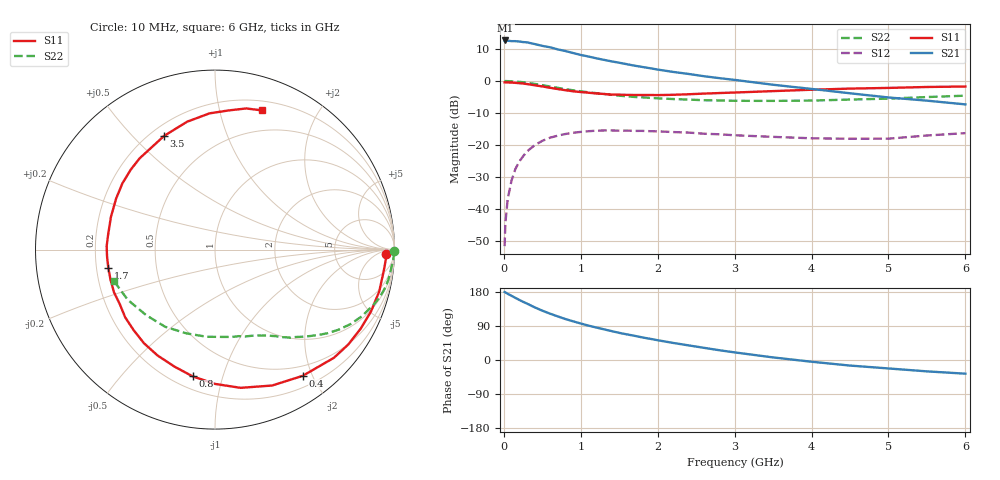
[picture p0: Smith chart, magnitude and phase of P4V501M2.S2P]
! SIEMENS Small Signal Semiconductors
! BFP182
! Si NPN RF Bipolar Junction Transistor in SOT143
! VCE = 0.5 V  IC = 1.2 mA
! Common Emitter S-Parameters:  March  1996
# GHz  S  MA  R  50
!  f  S11  S21  S12  S22
! GHz  MAG  ANG  MAG  ANG  MAG  ANG  MAG  ANG
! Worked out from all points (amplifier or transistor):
!   36 points, 10 MHz to 6 GHz, reference 50 ohm
!   highest |S21| = 12.7 dB at 20 MHz (marker M1)
!   |S21| within 3 dB of that: start of sweep to 740.6 MHz
!   unconditionally stable (mu >= 1): 2.31 GHz to end of sweep
!   at 250 MHz: K = 0.11, MSG = 17.9 dB, |S12| = -23.6 dB
!   at 1.4 GHz: K = 0.62, MSG = 10.8 dB, |S12| = -15.5 dB
!   at 6 GHz: K = 1.39, MAG = 0.8 dB, |S12| = -16.3 dB
!   S11 on the Smith chart (normalised r, x): 10 MHz: 33, -16; 400 MHz: 0.35, -1.86; 800 MHz: 0.28, -0.80; 1.7 GHz: 0.25, -0.08; 3.5 GHz: 0.25, +0.62; 6 GHz: 0.29, +1.36
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0.01  0.9518 -1.4  4.228 179.3  0.0026 87.4  0.995 -0.6
0.02  0.954 -3.0  4.306 178.5  0.0059 88.5  0.9977 -1.4
0.05  0.9476 -7.2  4.265 174.7  0.0142 87.6  0.9942 -3.3
0.1  0.9444 -14.3  4.198 169.4  0.0277 81.6  0.9863 -6.5
0.15  0.9349 -21.6  4.198 164.0  0.0419 76.3  0.9806 -9.9
0.25  0.9115 -35.5  4.065 153.6  0.0663 68.1  0.9557 -16.1
0.3  0.8958 -42.3  4.022 149.0  0.0788 64.1  0.9373 -18.9
0.4  0.8564 -55.2  3.784 139.0  0.0988 56.0  0.8997 -24.3
0.5  0.8215 -67.2  3.542 130.2  0.1157 49.0  0.8607 -28.9
0.6  0.7833 -79.5  3.368 122.3  0.1294 43.1  0.82 -33.0
0.8  0.7171 -100.0  2.944 108.1  0.148 32.3  0.7456 -39.7
0.9  0.6899 -109.1  2.739 102.1  0.1548 27.8  0.7145 -42.4
1.1  0.6548 -127.2  2.414 90.7  0.1636 20.2  0.6646 -47.1
1.4  0.6115 -150.0  2.027 76.3  0.1684 10.6  0.6089 -53.3
1.7  0.6032 -170.2  1.735 63.8  0.1655 4.1  0.5618 -58.4
1.9  0.6039 178.1  1.584 56.0  0.1638 0.4  0.544 -61.8
2.2  0.6076 162.7  1.386 45.1  0.1587 -3.8  0.5215 -67.1
2.8  0.6473 136.4  1.108 25.8  0.1465 -9.5  0.4959 -78.9
3.5  0.6941 114.1  0.873 6.8  0.1335 -10.9  0.4879 -95.5
4.5  0.7597 92.3  0.642 -14.7  0.1247 -7.0  0.512 -122.9
5.5  0.8055 77.5  0.492 -30.0  0.1402 0.5  0.5604 -149.9
6  0.819 71.2  0.43 -36.1  0.1527 -0.1  0.5893 -162.5
